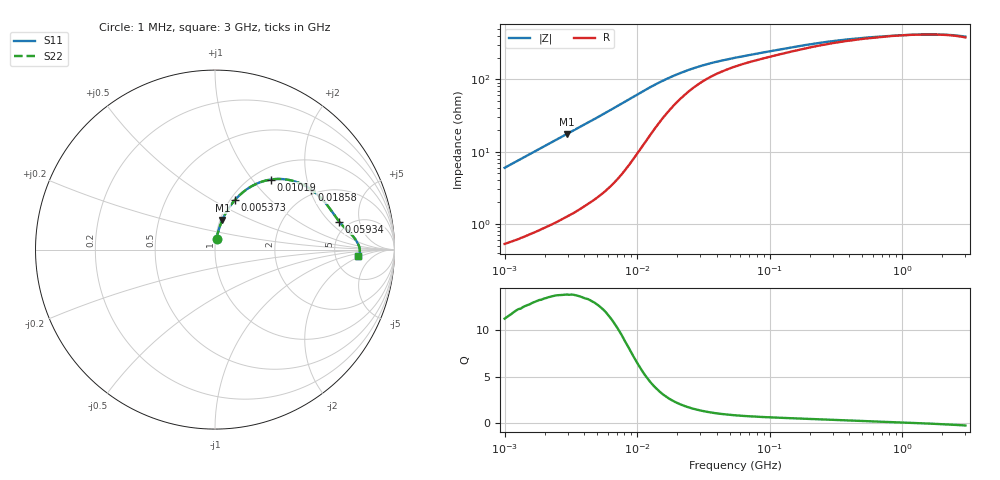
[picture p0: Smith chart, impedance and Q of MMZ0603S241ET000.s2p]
! S-Parameter Data Generated by TDK Corporation
! Copyright(C) 2025 TDK Corporation.
! All Rights Reserved.
! TDK P/N: MMZ0603S241ET000 (Chip Bead)
! Property: |Z|=240ohm at 100MHz
! Size(LxWxT): 0.6x0.3x0.3mm
! Model Type: s2p (Touchstone File Format Version 1.0)
! Frequency: DC=Yes Start=1MHz Stop=3000MHz 202points Log-sweep
! Model Generated on Feb. 6, 2025
! Terms and conditions regarding TDK Simulation Models:
! 1)This simulation model is being provided solely for informational
!  purposes. Please refer to the specifications of the products in
!  terms of detailed characteristics of such products.
! 2)In no event shall TDK Corporation of any of its subsidiaries be
!  liable for any loss or damage arising, directly or indirectly,
!  from any information contained in this simulation model, including,
!  but not limited to loss or damages arising from any inaccuracies,
!  omissions or errors in connection with such information.
! 3)Any and all copyrights on this simulation model are owned by
!  TDK Corporation.  Duplication or redistribution of this simulation
!  model without prior written permission from TDK Corporation
!  is prohibited.
! 4)This simulation model is subject to any modification or change
!  without any prior notice.
! 5)Neither TDK Corporation nor any of its subsidiaries shall make any
!  warranty, express or implied, including but not limited to the
!  correctness, implied warranties of merchantability and fitness for
!  a particular purpose with respect to this simulation models.
! 6)The use of this simulation model shall be deemed to have consented
!  to the terms and conditions hereof.
! Port Assignments:
!  1 ---@@@--- 2
! Applicable Conditions:
!  Temperature = 25 degC
!  DC Bias Current = 0 A
!  Small Signal Operation
# Hz S MA R 50
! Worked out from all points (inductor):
!   201 points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, 1 MHz to 3 GHz, reference 50 ohm
!   read as one part in series: L = 948 nH near 1.041 MHz
!   highest Q = 13.8 at 2.947 MHz (marker M1), where L = 940 nH
!   self-resonance near 1.454 GHz
!   S11 on the Smith chart (normalised r, x): 1 MHz: 1.01, +0.12; 5.373 MHz: 1.05, +0.64; 10.19 MHz: 1.20, +1.24; 18.58 MHz: 1.84, +2.05; 59.34 MHz: 4.15, +2.61; 3 GHz: 8.61, -1.72
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1000000  0.05942 81.5  0.993 -3.4  0.993 -3.4  0.05942 81.5
1751453  0.103 79.8  0.9869 -5.9  0.9869 -5.9  0.103 79.8
2947212  0.1699 76.1  0.9733 -9.8  0.9733 -9.8  0.1699 76.1
3900413  0.2215 73.0  0.959 -12.8  0.959 -12.8  0.2215 73.0
5372736  0.2977 68.1  0.931 -17.3  0.931 -17.3  0.2977 68.1
7400828  0.3937 61.1  0.8802 -23.1  0.8802 -23.1  0.3937 61.1
8686058  0.4469 56.6  0.8413 -26.3  0.8413 -26.3  0.4469 56.6
1.019448e7  0.499 51.5  0.792 -29.5  0.792 -29.5  0.499 51.5
1.196486e7  0.546 46.0  0.7344 -32.3  0.7344 -32.3  0.546 46.0
1.461624e7  0.593 39.2  0.6577 -34.7  0.6577 -34.7  0.593 39.2
1.858443e7  0.6324 31.8  0.5705 -35.8  0.5705 -35.8  0.6324 31.8
2.362996e7  0.6577 25.8  0.4979 -35.0  0.4979 -35.0  0.6577 25.8
2.886629e7  0.6723 21.7  0.4499 -33.5  0.4499 -33.5  0.6723 21.7
3.976269e7  0.6899 16.8  0.3935 -30.4  0.3935 -30.4  0.6899 16.8
5.477226e7  0.705 13.4  0.3543 -27.5  0.3543 -27.5  0.705 13.4
5.933785e7  0.7088 12.8  0.3461 -26.9  0.3461 -26.9  0.7088 12.8
2.136344e8  0.7694 5.9  0.2476 -18.6  0.2476 -18.6  0.7694 5.9
3.741707e8  0.7866 3.9  0.2216 -13.8  0.2216 -13.8  0.7866 3.9
8.005644e8  0.8011 1.7  0.2006 -6.8  0.2006 -6.8  0.8011 1.7
1.782824e9  0.8071 -0.6  0.1932 2.6  0.1932 2.6  0.8071 -0.6
2.359433e9  0.8055 -1.6  0.1961 6.5  0.1961 6.5  0.8055 -1.6
3e9  0.7992 -2.6  0.2048 10.1  0.2048 10.1  0.7992 -2.6
